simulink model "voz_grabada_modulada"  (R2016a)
settings: Solver=VariableStepAuto  StartTime=0.0  StopTime=10  RelTol=1e-3
undefined symbols (not defined in the file): DiscIntNeverNeededParam
libraries: dsparch4 x1, dspsnks4 x1, commsynccomp2 x1, dspsrcs4 x1

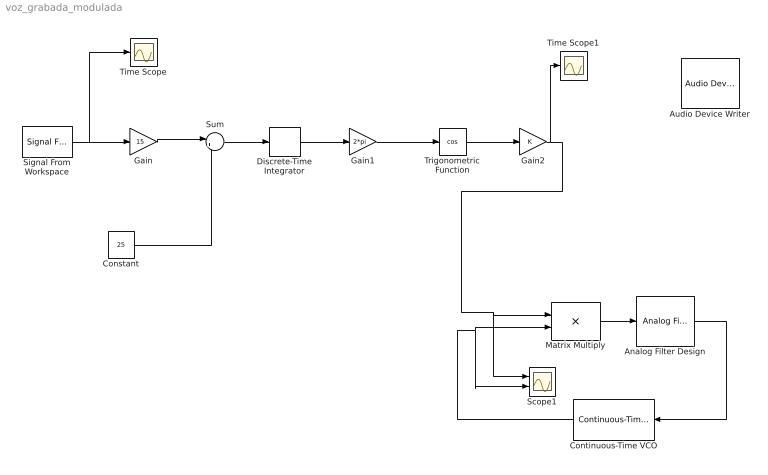
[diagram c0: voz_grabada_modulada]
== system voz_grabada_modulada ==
  Analog Filter Design : dsparch4/Analog Filter Design  method=Butterworth  filttype=Lowpass  N=5  Wlo=2*pi*10  Whi=80  Rp=2  Rs=40
  Audio Device Writer : dspsnks4/Audio Device Writer  Commented=on  Driver=DirectSound  Device=Default  InheritSampleRate=on  SampleRate=44100  BitDepth=16-bit integer  BufferSize=4096  NumBuffers=10  DefaultOutputChannelMapping=on  OutputChannelMapping=1:2  OutputNumUnderrunSamples=off  DriverIdx=1  DeviceWarnFlag=''
  Constant : Constant  Value=25
  Continuous-Time VCO : commsynccomp2/Continuous-Time VCO  Ac=1  Fc=100  Kc=50  Ph=0
  Discrete-Time Integrator : DiscreteIntegrator  InitialConditionSetting=State (most efficient)  SampleTime=-1  ICPrevOutput=DiscIntNeverNeededParam  ICPrevScaledInput=DiscIntNeverNeededParam
  Gain : Gain  Gain=15
  Gain1 : Gain  Gain=2*pi
  Gain2 : Gain
  Matrix Multiply : Product  Multiplication=Matrix(*)
  Scope1 : Scope  NumInputPorts=2
  Signal From Workspace : dspsrcs4/Signal From Workspace  X=mySpeech  Ts=1/20000  nsamps=10000  OutputAfterFinalValue=Setting to zero  ignoreOrWarnInputAndFrameLengths=off  OutputFrames=off
  Sum : Sum  Inputs=|++
  Time Scope : Scope
  Time Scope1 : Scope
  Trigonometric Function : Trigonometry  Operator=cos
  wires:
  Gain/1 -> Sum/1
  Constant/1 -> Sum/2
  Gain1/1 -> Trigonometric Function/1
  Trigonometric Function/1 -> Gain2/1
  Sum/1 -> Discrete-Time Integrator/1
  Discrete-Time Integrator/1 -> Gain1/1
  Signal From Workspace/1 -> Time Scope/1, Gain/1
  Gain2/1 -> Time Scope1/1, Matrix Multiply/1, Scope1/1
  Matrix Multiply/1 -> Analog Filter Design/1
  Analog Filter Design/1 -> Continuous-Time VCO/1
  Continuous-Time VCO/1 -> Matrix Multiply/2, Scope1/2
